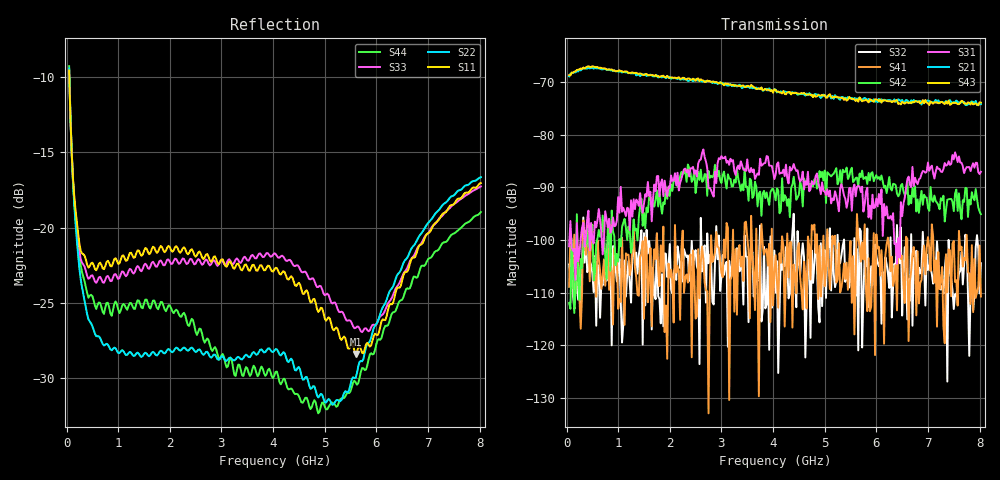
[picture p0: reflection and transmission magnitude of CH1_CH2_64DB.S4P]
!Agilent Technologies,E5071C,MY46316741,A.11.02
!Date: Thu May 28 14:29:24 2026
!Data & Calibration Information:
!1:CH1 INPUT 2:CH1 OUTPUT 3:CH2 INPUT 4:CH2 OUTPUT
!Freq	S11:SOLT4(ON)	S12:SOLT4(ON)	S13:SOLT4(ON)	S14:SOLT4(ON)
!	S21:SOLT4(ON)	S22:SOLT4(ON)	S23:SOLT4(ON)	S24:SOLT4(ON)
!	S31:SOLT4(ON)	S32:SOLT4(ON)	S33:SOLT4(ON)	S34:SOLT4(ON)
!	S41:SOLT4(ON)	S42:SOLT4(ON)	S43:SOLT4(ON)	S44:SOLT4(ON)
!PortZ  Port1:50+j0  Port2:50+j0  Port3:50+j0  Port4:50+j0
!Above PortZ is port z conversion or system Z0 setting when saving the data.
!When reading, reference impedance value at option line is always used.
# Hz S dB R 50
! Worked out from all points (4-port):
!   320 points, 50 MHz to 8.025 GHz, reference 50 ohm
!   strongest paths, dB at 50 MHz, 2.05 GHz, 4.05 GHz, 6.05 GHz, 8.025 GHz:
!     S43: -68.7, -69.1, -71.5, -73.7, -73.9
!     S21: -69.0, -69.2, -71.5, -73.2, -74.2
!     S31: -101.2, -88.8, -87.6, -91.3, -87.1
!     S42: -112.0, -90.7, -92.5, -88.1, -95.1
!     S41: -108.9, -107.7, -102.9, -101.3, -110.7
!     S32: -104.7, -110.1, -110.0, -105.0, -104.4
!   lowest |S11| = -28.4 dB at 5.6 GHz (marker M1), VSWR 1.08, Z = 48.1 - j3.24 ohm
!   |S11| at or under -10 dB: 53.38 MHz to end of sweep
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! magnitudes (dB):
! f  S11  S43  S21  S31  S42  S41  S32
! 50 MHz  -9.6  -68.7  -69.0  -101.2  -112.0  -108.9  -104.7
! 125 MHz  -16.7  -68.3  -68.3  -102.1  -106.6  -106.2  -110.4
! 275 MHz  -21.6  -67.5  -67.8  -99.8  -103.6  -116.8  -114.4
! 725 MHz  -22.8  -67.4  -67.5  -99.7  -98.8  -103.7  -104.6
! 4.025 GHz  -22.8  -71.4  -71.4  -88.4  -91.2  -106.4  -102.0
! 5.6 GHz  -28.4  -73.6  -73.2  -91.7  -88.2  -107.0  -110.6
! 8.025 GHz  -17.0  -73.9  -74.2  -87.1  -95.1  -110.7  -104.4
